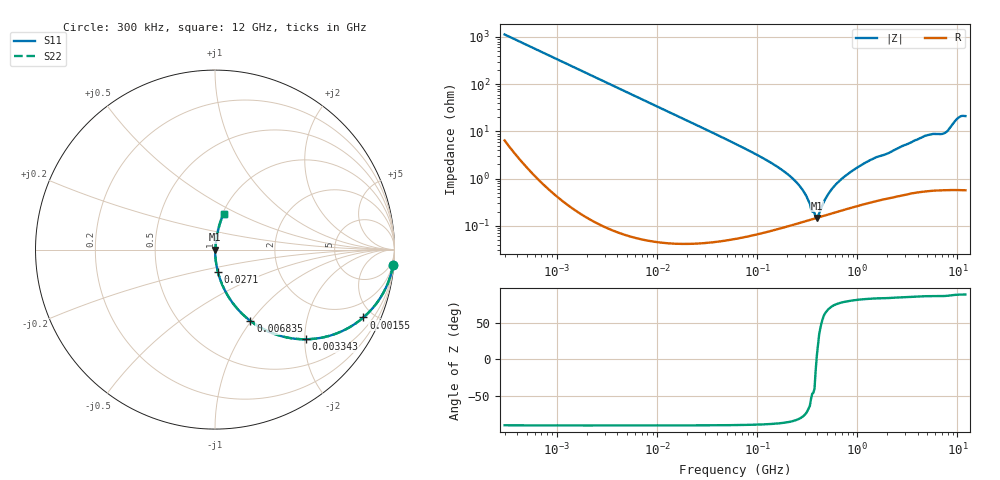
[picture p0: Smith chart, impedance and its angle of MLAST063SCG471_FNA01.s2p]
! MLAST063SCG471_FNA01  S-PARAMETER MODEL  ( General Type )
! Model Generated by TAIYO YUDEN Corporation (http://www.ty-top.com)
! Version 1.0
! TAIYO YUDEN Control No. 160830
! Copyright(c) 2016 TAIYO YUDEN CO.,LTD. All Rights Reserved.
! Product Description (link to TY-COMPAS)
! https://ds.yuden.co.jp/TYCOMPAS/or/detail?pn=MLAST063SCG471JFNA01&u=M
! Products Name : Multilayer Ceramic Capacitors
! Characteristics :
!  Capacitance : 470 pF , Rated Voltage : 25V , TCC : CG / C0G
!  Case Size : 0.6 x 0.3 / 0.024 x 0.012 [mm/inch] , Thickness : 0.3 / 0.012 [mm/inch]
!  (Conditions: Temperature = 25 degC , DC Bias Current/Voltage = 0A / 0V)
! External Node Assignments :
!  1  o---| |---o  2
! GND o---------o GND
! Frequency Range : 0.3MHz  -  12000MHz  [ 401 STEP ]
# MHz S RI R 50
! Freq[MHz].  S11 Real  S11 Imag  S21 Real  S21 Imag  S12 Real  S12 Imag  S22 Real  S22 Imag
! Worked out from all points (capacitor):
!   401 points, 300 kHz to 12 GHz, reference 50 ohm
!   read as one part in series: C = 470 pF near 316.3 kHz
!   lowest |Z| = 147 mohm at 393.6 MHz (marker M1)
!   series resonance near 391.3 MHz, so ESL is about 350 pH
!   S11 on the Smith chart (normalised r, x): 300 kHz: 1, -23; 1.55 MHz: 1.00, -4.37; 3.343 MHz: 1.00, -2.03; 6.835 MHz: 1.00, -0.99; 27.1 MHz: 1.00, -0.25; 12 GHz: 1.01, +0.42
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0.3  0.9917 -0.0878  0.00828 0.0878  0.00828 0.0878  0.9917 -0.0878
0.799488  0.9469 -0.2235  0.0531 0.2235  0.0531 0.2235  0.9469 -0.2235
1.550389  0.8265 -0.3782  0.1735 0.3782  0.1735 0.3782  0.8265 -0.3782
1.769972  0.7852 -0.4102  0.2148 0.4102  0.2148 0.4102  0.7852 -0.4102
3.342642  0.5064 -0.4995  0.4936 0.4995  0.4936 0.4995  0.5064 -0.4995
6.834849  0.1972 -0.3974  0.8028 0.3974  0.8028 0.3974  0.1972 -0.3974
10.44266  0.0954 -0.293  0.9046 0.293  0.9046 0.293  0.0954 -0.293
27.10171  0.0156 -0.1224  0.9844 0.1224  0.9844 0.1224  0.0156 -0.1224
60  0.00355 -0.0549  0.9965 0.0549  0.9965 0.0549  0.00355 -0.0549
132.8329  0.00127 -0.0225  0.9987 0.0225  0.9987 0.0225  0.00127 -0.0225
213.9924  0.00113 -0.0111  0.9989 0.0111  0.9989 0.0111  0.00113 -0.0111
286.3882  0.00123 -0.00546  0.9988 0.00546  0.9988 0.00546  0.00123 -0.00546
353.9943  0.00137 -0.00146  0.9986 0.00146  0.9986 0.00146  0.00137 -0.00146
393.5654  0.00147 0.000113  0.9985 -0.000113  0.9985 -0.000113  0.00147 0.000113
526.7124  0.00179 0.00478  0.9982 -0.00478  0.9982 -0.00478  0.00179 0.00478
704.9044  0.00221 0.00976  0.9978 -0.00976  0.9978 -0.00976  0.00221 0.00976
1197.383  0.00334 0.0212  0.9967 -0.0212  0.9967 -0.0212  0.00334 0.0212
2088.533  0.00504 0.0348  0.995 -0.0348  0.995 -0.0348  0.00504 0.0348
4747.894  0.0116 0.0791  0.9884 -0.0791  0.9884 -0.0791  0.0116 0.0791
7448.838  0.0139 0.0904  0.9861 -0.0904  0.9861 -0.0904  0.0139 0.0904
10236.47  0.042 0.1864  0.958 -0.1864  0.958 -0.1864  0.042 0.1864
12000  0.0475 0.1997  0.9525 -0.1997  0.9525 -0.1997  0.0475 0.1997
